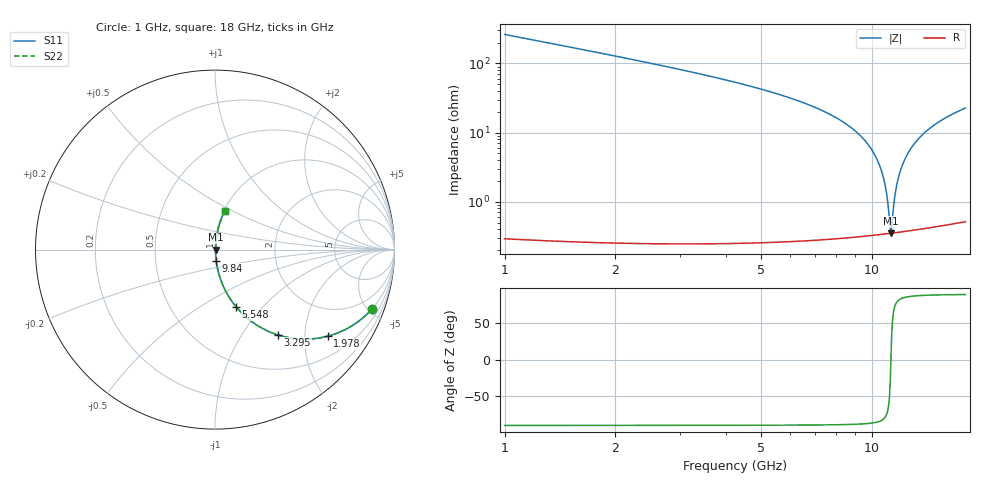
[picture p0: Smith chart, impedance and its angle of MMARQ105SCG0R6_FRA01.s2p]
! MMARQ105SCG0R6_FRA01  S-PARAMETER MODEL  ( General Type )
! Model Generated by TAIYO YUDEN Corporation (http://www.ty-top.com)
! Version 1.0
! TAIYO YUDEN Control No. 200326
! Copyright(c) 2020 TAIYO YUDEN CO.,LTD. All Rights Reserved.
! Product Description (link to TY-COMPAS)
! https://ds.yuden.co.jp/TYCOMPAS/or/detail?pn=MMARQ105SCG0R6BFRA01&u=M
! Products Name : Multilayer Ceramic Capacitors
! Characteristics :
!  Capacitance : 0.6 pF , Rated Voltage : 250V , TCC : CG / C0G
!  Case Size : 1.0 x 0.5 / 0.039 x 0.02 [mm/inch] , Thickness : 0.5 / 0.02 [mm/inch]
!  (Conditions: Temperature = 25 degC , DC Bias Current/Voltage = 0A / 0V)
! External Node Assignments :
!  1  o---| |---o  2
! GND o---------o GND
! Frequency Range : 1GHz  -  18GHz  [ 401 STEP ]
# MHz S RI R 50
! Freq[MHz].  S11 Real  S11 Imag  S21 Real  S21 Imag  S12 Real  S12 Imag  S22 Real  S22 Imag
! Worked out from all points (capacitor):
!   401 points, 1 GHz to 18 GHz, reference 50 ohm
!   read as one part in series: C = 602 fF near 1.085 GHz
!   lowest |Z| = 351 mohm at 11.29 GHz (marker M1)
!   series resonance near 11.28 GHz, so ESL is about 330 pH
!   S11 on the Smith chart (normalised r, x): 1 GHz: 1.01, -5.25; 1.978 GHz: 1.01, -2.59; 3.295 GHz: 1.00, -1.47; 5.548 GHz: 1.01, -0.72; 9.84 GHz: 1.01, -0.13; 18 GHz: 1.01, +0.45
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1000  0.873 -0.3324  0.127 0.3324  0.127 0.3324  0.873 -0.3324
1977.5  0.6269 -0.4827  0.3731 0.4827  0.3731 0.4827  0.6269 -0.4827
3295  0.3509 -0.4756  0.6491 0.4756  0.6491 0.4756  0.3509 -0.4756
3847.5  0.2705 -0.4422  0.7295 0.4422  0.7295 0.4422  0.2705 -0.4422
5547.5  0.1174 -0.3183  0.8826 0.3183  0.8826 0.3183  0.1174 -0.3183
6695  0.0637 -0.239  0.9363 0.239  0.9363 0.239  0.0637 -0.239
8352.5  0.0228 -0.1394  0.9772 0.1394  0.9772 0.1394  0.0228 -0.1394
9500  0.0096 -0.0799  0.9904 0.0799  0.9904 0.0799  0.0096 -0.0799
9840  0.00729 -0.0636  0.9927 0.0636  0.9927 0.0636  0.00729 -0.0636
10350  0.00493 -0.0401  0.9951 0.0401  0.9951 0.0401  0.00493 -0.0401
10732.5  0.00392 -0.0232  0.9961 0.0232  0.9961 0.0232  0.00392 -0.0232
10987.5  0.00358 -0.0123  0.9964 0.0123  0.9964 0.0123  0.00358 -0.0123
11200  0.00349 -0.0034  0.9965 0.0034  0.9965 0.0034  0.00349 -0.0034
11285  0.00349 0.000121  0.9965 -0.000121  0.9965 -0.000121  0.00349 0.000121
11370  0.00352 0.00361  0.9965 -0.00361  0.9965 -0.00361  0.00352 0.00361
11540  0.00365 0.0105  0.9963 -0.0105  0.9963 -0.0105  0.00365 0.0105
11710  0.00388 0.0173  0.9961 -0.0173  0.9961 -0.0173  0.00388 0.0173
11965  0.00438 0.0273  0.9956 -0.0273  0.9956 -0.0273  0.00438 0.0273
12347.5  0.00548 0.0419  0.9945 -0.0419  0.9945 -0.0419  0.00548 0.0419
13452.5  0.0107 0.0816  0.9893 -0.0816  0.9893 -0.0816  0.0107 0.0816
15195  0.0237 0.1375  0.9763 -0.1375  0.9763 -0.1375  0.0237 0.1375
18000  0.0532 0.2134  0.9468 -0.2134  0.9468 -0.2134  0.0532 0.2134
